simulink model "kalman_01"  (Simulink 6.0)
settings: Solver=FixedStepDiscrete  StartTime=0.0  StopTime=50.0  FixedStep=1  RelTol=1e-3
libraries: dspadpt3 x1

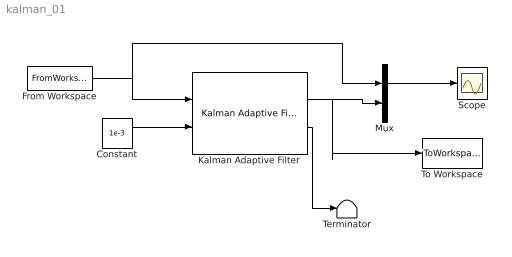
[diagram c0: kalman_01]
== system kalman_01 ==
  Constant : Constant  Value=1e-3
  From Workspace : FromWorkspace  VariableName=[tout,x_accel]  SampleTime=1
  Kalman Adaptive Filter : dspadpt3/Kalman Adaptive Filter  Ntaps=50  Jmin=0.0077  q=0.1  ic0=0  K0=0.5  Adapt=off  RstPort=None
  Mux : Mux  Inputs=2
  Scope : Scope
  Terminator : Terminator
  To Workspace : ToWorkspace  VariableName=simout  SampleTime=-1  SaveFormat=Array
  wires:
  From Workspace/1 -> Mux/1, Kalman Adaptive Filter/1
  Mux/1 -> Scope/1
  Kalman Adaptive Filter/1 -> Mux/2, To Workspace/1
  Constant/1 -> Kalman Adaptive Filter/2
  Kalman Adaptive Filter/2 -> Terminator/1
